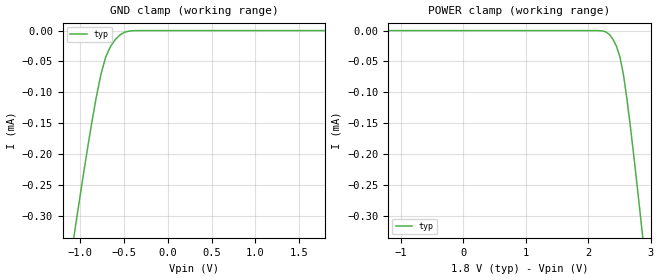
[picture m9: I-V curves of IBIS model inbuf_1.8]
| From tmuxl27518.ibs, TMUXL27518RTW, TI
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| inbuf_1.8
[Model]   inbuf_1.8
Model_type   Input
Vinl = 0.39
Vinh = 0.77
|   typ   min   max
C_comp   2.533030e-13   NA   NA
[Voltage Range]   1.8   NA   NA
[Temperature Range]   27   NA   NA
[Power Clamp Reference]   1.8   NA   NA
[GND Clamp Reference]   0   NA   NA
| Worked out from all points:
|   GND clamp passes 1 mA (typ) near -1.75 V on its own axis
[GND Clamp]
|   Voltage   I(typ)   I(min)   I(max)
-3.6V     -2.904mA   NA         NA
-1.091V   -350.8uA   NA         NA
-1.036V   -299.3uA   NA         NA
-872.7mV  -152.5uA   NA         NA
-818.2mV  -108.6uA   NA         NA
-763.6mV  -70.55uA   NA         NA
-709.1mV  -42.64uA   NA         NA
-654.5mV  -25.68uA   NA         NA
-545.5mV  -6.858uA   NA         NA
-490.9mV  -2.484uA   NA         NA
-381.8mV  -148.1nA   NA         NA
1.8V      124.9pA    NA         NA
[POWER Clamp]
|   Voltage   I(typ)   I(min)   I(max)
-1.8V     31.34nA    NA         NA
2.127V    -27.93nA   NA         NA
2.291V    -2.484uA   NA         NA
2.4V      -14.53uA   NA         NA
2.455V    -25.68uA   NA         NA
2.509V    -42.64uA   NA         NA
2.564V    -70.55uA   NA         NA
2.618V    -108.6uA   NA         NA
2.673V    -152.5uA   NA         NA
2.836V    -299.3uA   NA         NA
2.891V    -350.8uA   NA         NA
3.6V      -1.054mA   NA         NA
